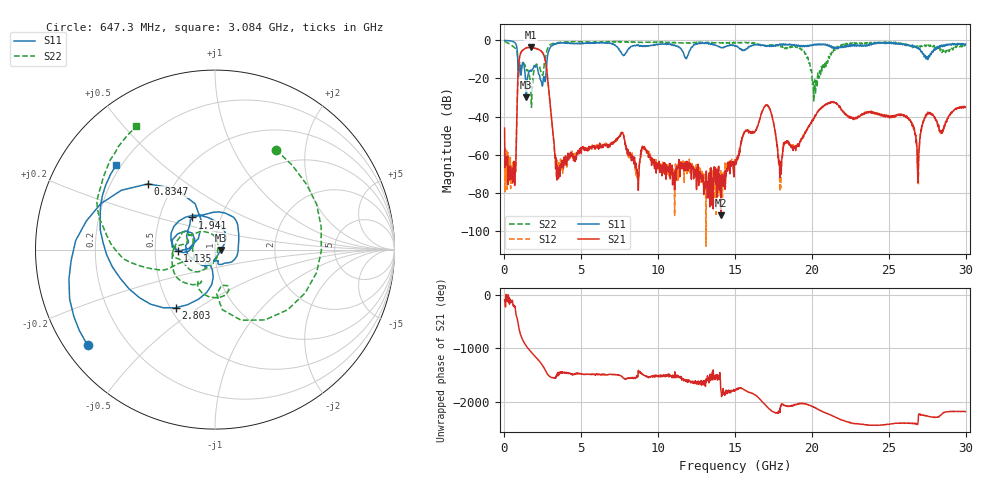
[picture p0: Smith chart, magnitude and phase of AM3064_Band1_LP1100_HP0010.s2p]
# Hz S DB R 50.0
!freq dBS11 angS11 dBS21 angS21 dBS12 angS12 dBS22 angS22
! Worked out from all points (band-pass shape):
!   1600 points, 10 MHz to 29.98 GHz, reference 50 ohm
!   highest |S21| = -3.63 dB at 1.716 GHz (marker M1); lowest = -91.8 dB at 14.09 GHz (marker M2)
!   |S21| within 3 dB of the highest: 1.056 GHz to 2.493 GHz (1.437 GHz wide, 81 % of centre)
!   lowest |S11| = -29.9 dB at 1.416 GHz (marker M3), VSWR 1.07, Z = 53.3 - j0.232 ohm
!   |S11| at or under -10 dB: 866 MHz to 2.775 GHz (1.909 GHz wide, 105 % of centre); 27.52415 GHz to 27.53311 GHz (8.959 MHz wide, 0.0325 % of centre)
!   |S22| runs from -35.2 to -0.4 dB; largest |S21 - S12| = 0.0086
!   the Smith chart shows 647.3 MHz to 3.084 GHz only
!   S11 on the Smith chart (normalised r, x): 647.3 MHz: 0.07, -0.33; 834.7 MHz: 0.36, +0.36; 1.135 GHz: 0.66, -0.01; 1.941 GHz: 0.73, +0.28; 2.803 GHz: 0.53, -0.41; 3.084 GHz: 0.18, +0.36
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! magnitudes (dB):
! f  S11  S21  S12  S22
! 10 MHz  0.0  -46.1  -58.1  -0.4
! 647.3 MHz  -1.0  -64.0  -65.5  -3.7
! 834.7 MHz  -5.6  -30.6  -30.4  -7.5
! 1.135 GHz  -13.7  -5.6  -5.5  -13.3
! 1.416 GHz  -29.9  -3.9  -3.9  -15.7
! 1.716 GHz  -15.8  -3.6  -3.7  -25.9
! 1.941 GHz  -13.2  -4.0  -4.0  -15.4
! 2.803 GHz  -8.2  -19.4  -19.4  -4.3
! 3.084 GHz  -2.8  -43.2  -43.0  -1.7
! 3.478 GHz  -1.6  -66.9  -68.8  -1.1
! 5.015 GHz  -1.5  -57.2  -56.4  -0.6
! 7.62 GHz  -6.9  -48.5  -48.3  -0.7
! 10 GHz  -2.1  -64.9  -64.6  -1.0
! 14.09 GHz  -3.8  -91.8  -70.3  -1.3
! 15 GHz  -2.9  -63.8  -63.9  -1.5
! 17.01 GHz  -3.1  -34.1  -33.9  -2.9
! 17.93 GHz  -2.0  -72.0  -72.8  -2.8
! 19.99 GHz  -2.8  -42.3  -42.4  -18.2
! 25 GHz  -1.1  -39.9  -39.7  -1.2
! 26.89 GHz  -3.8  -74.8  -69.4  -3.3
! 27.49 GHz  -8.6  -38.6  -38.6  -2.8
! 29.98 GHz  -1.9  -35.2  -35.0  -2.9
